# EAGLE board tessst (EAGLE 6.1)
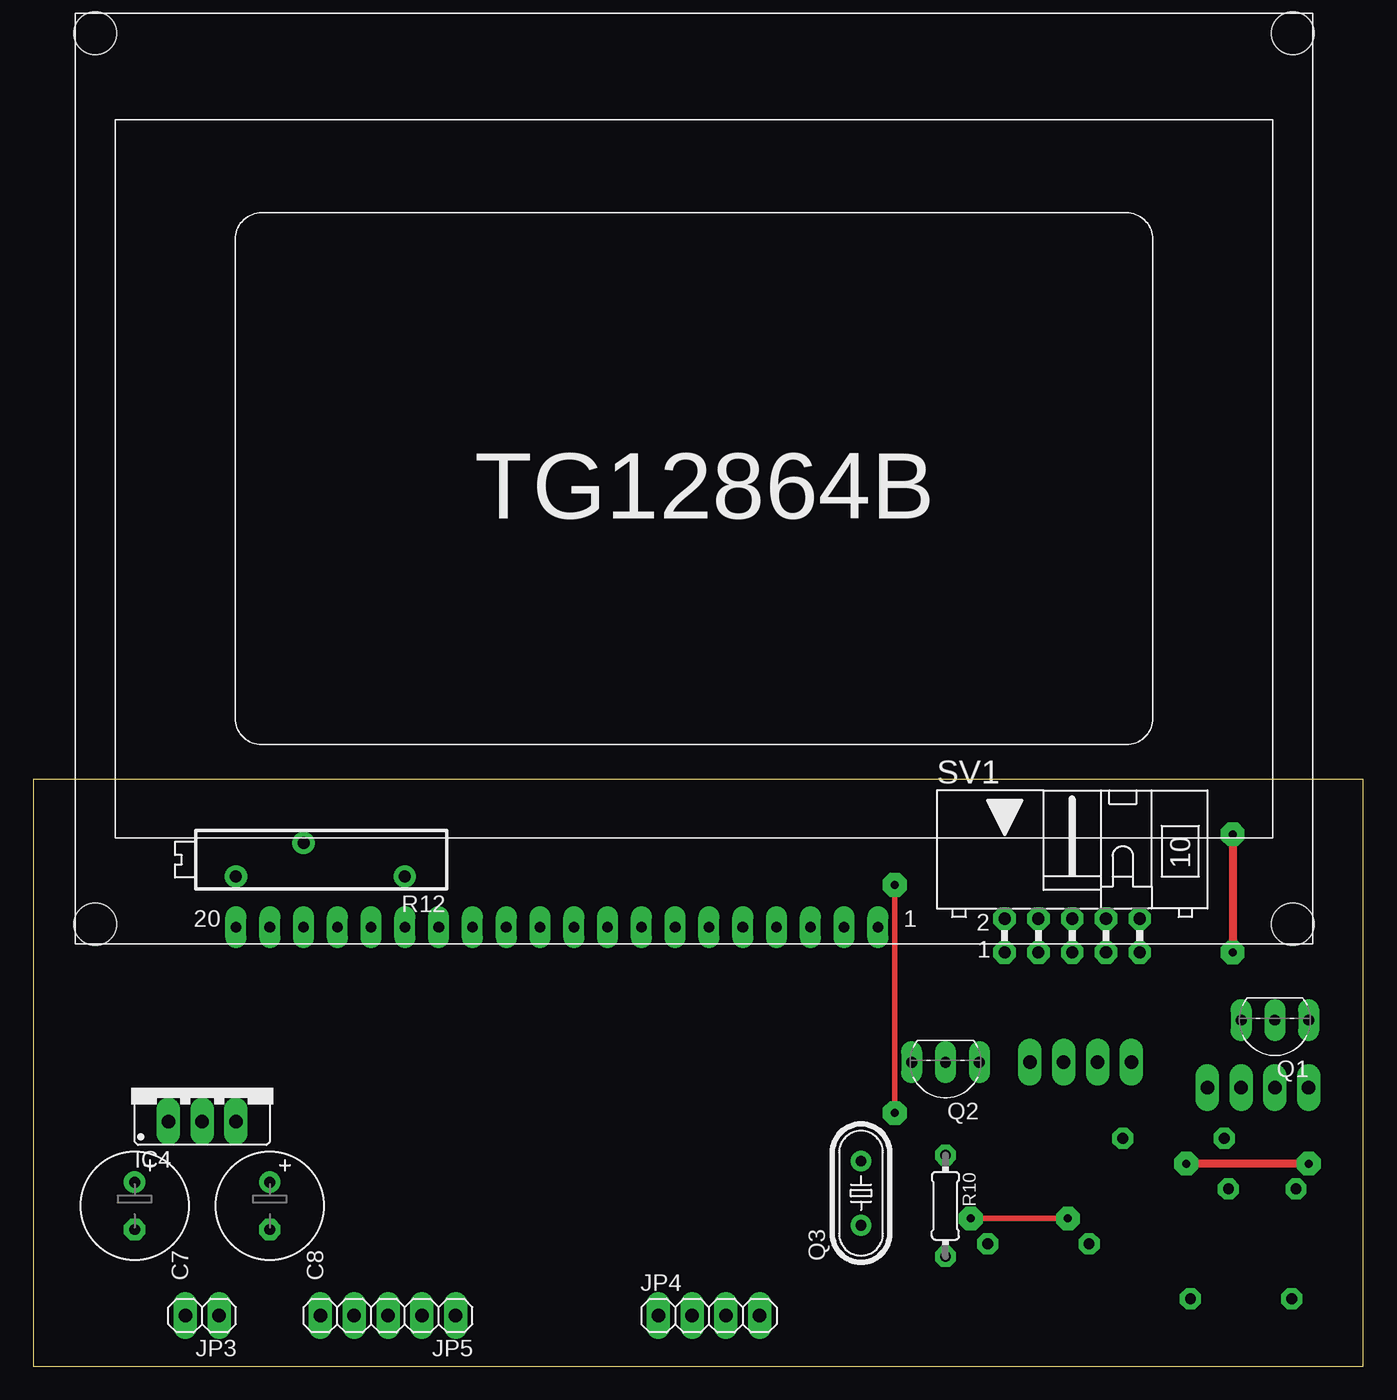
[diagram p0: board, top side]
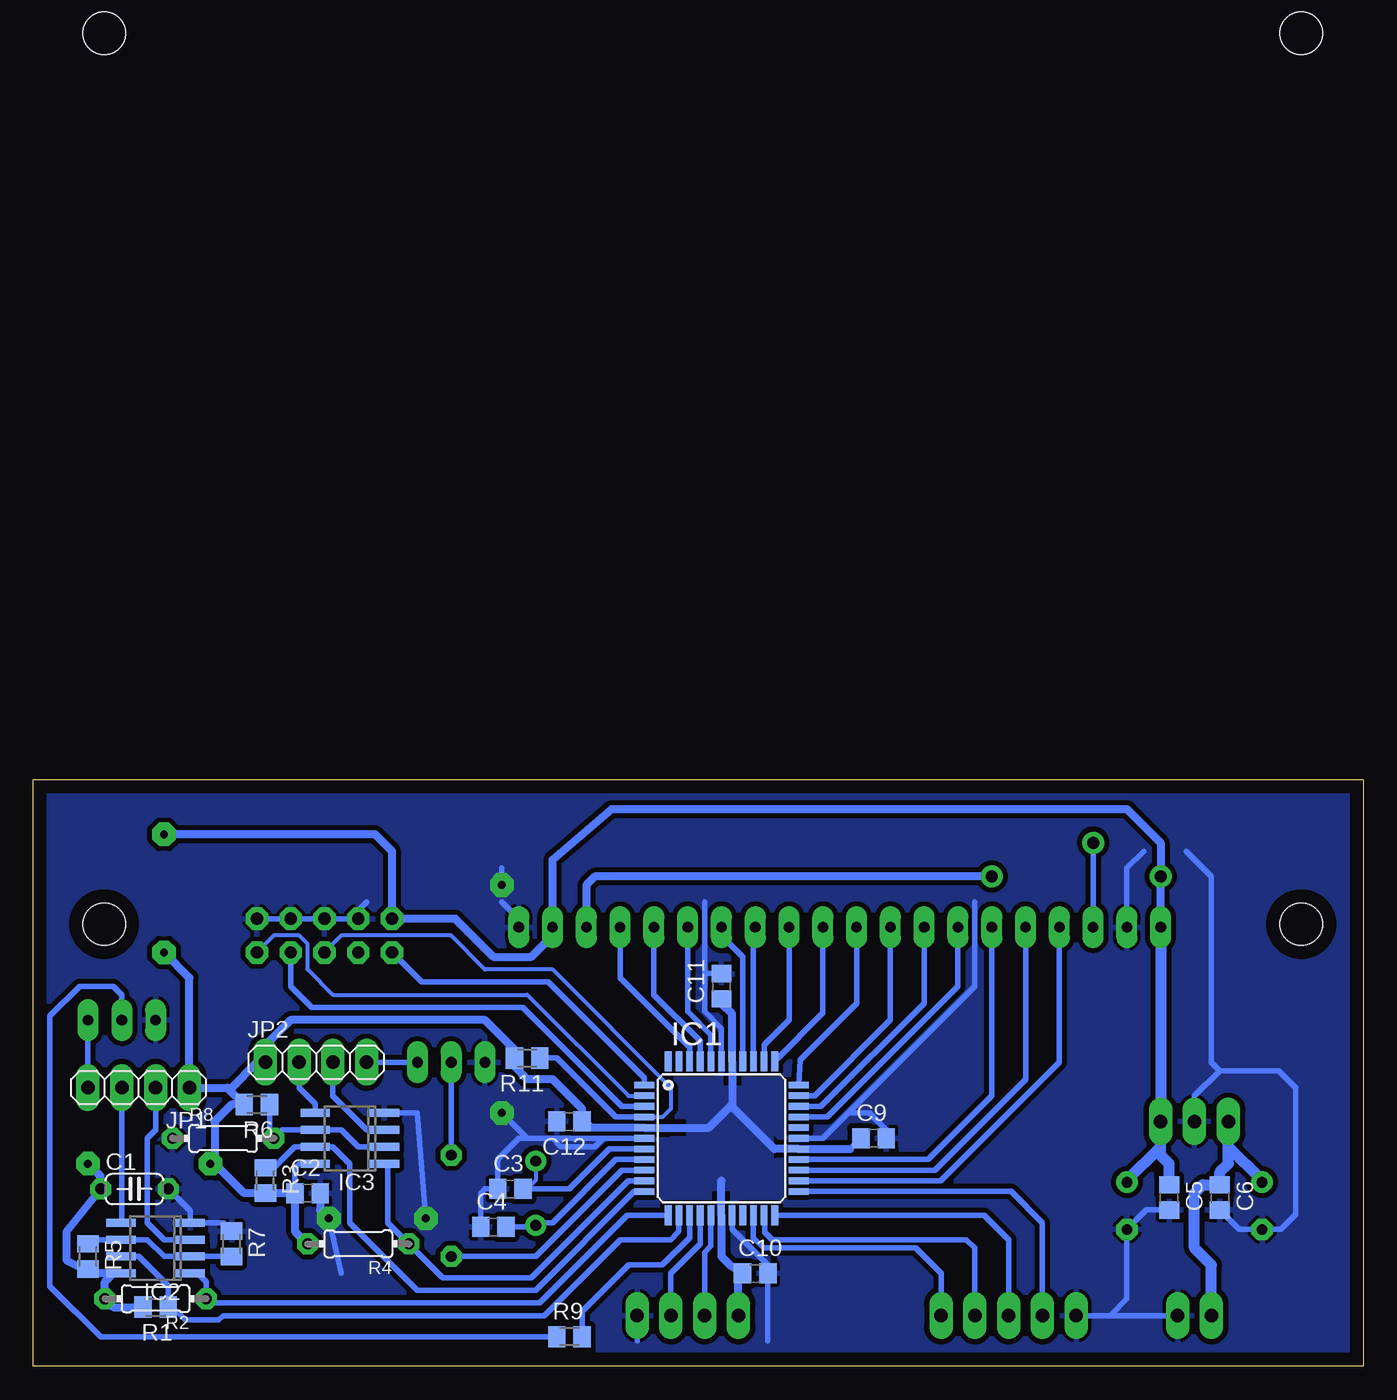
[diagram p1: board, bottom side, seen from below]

Size 100 x 44.12 mm. Coordinates in mm from the lower left corner, seen from the top.
Outline: 0,0 100,0 100,44.12 0,44.12 0,0
Copper layers (1*16): Top 0.035mm / dielectric 1.5mm / Bottom 0.035mm
Design rules: minimum track width 10mil, minimum drill 24mil, track to track 15mil, track to pad 15mil, pad to pad 8mil, via to via 8mil, smd to smd 8mil, copper to edge 40mil, drill to drill 8mil, minimum pad ring 15mil, minimum via ring 15mil, stop-mask expansion 4mil, vias tented up to drill 0mil, thermal gap 10mil

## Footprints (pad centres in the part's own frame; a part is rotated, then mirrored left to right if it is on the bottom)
C050-024X044 = drill 0.813 octagon: 1 -2.54,0; 2 2.54,0
C0805 = smd 1.3 x 1.5: 1 -0.95,0; 2 0.95,0
E3,5-8 = drill 0.813 pad 1.6: + -1.778,0 | drill 0.813 pad 1.6 octagon: - 1.778,0
TQFP44 = smd 1.5 x 0.5: 1 -5.8,4; 2 -5.8,3.2; 3 -5.8,2.4; 4 -5.8,1.6; 5 -5.8,0.8; 6 -5.8,0; 7 -5.8,-0.8; 8 -5.8,-1.6; 9 -5.8,-2.4; 10 -5.8,-3.2; 11 -5.8,-4; 23 5.8,-4; 24 5.8,-3.2; 25 5.8,-2.4; 26 5.8,-1.6; 27 5.8,-0.8; 28 5.8,0; 29 5.8,0.8; 30 5.8,1.6; 31 5.8,2.4; 32 5.8,3.2; 33 5.8,4 | smd 0.5 x 1.5: 12 -4,-5.8; 13 -3.2,-5.8; 14 -2.4,-5.8; 15 -1.6,-5.8; 16 -0.8,-5.8; 17 0,-5.8; 18 0.8,-5.8; 19 1.6,-5.8; 20 2.4,-5.8; 21 3.2,-5.8; 22 4,-5.8; 34 4,5.8; 35 3.2,5.8; 36 2.4,5.8; 37 1.6,5.8; 38 0.8,5.8; 39 0,5.8; 40 -0.8,5.8; 41 -1.6,5.8; 42 -2.4,5.8; 43 -3.2,5.8; 44 -4,5.8
SO08 = smd 0.6 x 2.2: 1 -1.905,-2.6; 2 -0.635,-2.6; 3 0.635,-2.6; 4 1.905,-2.6; 5 1.905,2.6; 6 0.635,2.6; 7 -0.635,2.6; 8 -1.905,2.6
78XXS = drill 1.016 long: GND 0,-2.54; IN -2.54,-2.54; OUT 2.54,-2.54
1X04 = drill 1.016 long: 1 -3.81,0; 2 -1.27,0; 3 1.27,0; 4 3.81,0
1X02 = drill 1.016 long: 1 -1.27,0; 2 1.27,0
1X05 = drill 1.016 long: 1 -5.08,0; 2 -2.54,0; 3 0,0; 4 2.54,0; 5 5.08,0
TO92-EBC = drill 0.813 long: B 0,-1.27; C -2.54,-1.27; E 2.54,-1.27
HC49/S = drill 0.813: 1 -2.413,0; 2 2.413,0
M0805 = smd 1.3 x 1.6: 1 -0.95,0; 2 0.95,0
0204/7 = drill 0.813 octagon: 1 -3.81,0; 2 3.81,0
RTRIMT18 = drill 0.9: 1 -7.62,1.27; 2 0,-1.27; 3 5.08,1.27
ML10L = drill 0.914 octagon: 1 -5.08,-1.27; 2 -5.08,1.27; 3 -2.54,-1.27; 4 -2.54,1.27; 5 0,-1.27; 6 0,1.27; 7 2.54,-1.27; 8 2.54,1.27; 9 5.08,-1.27; 10 5.08,1.27
TG12864B = drill 0.8 long: /RST 19.685,1.27; CS1 24.765,1.27; CS2 22.225,1.27; D/I 52.705,1.27; DB0 45.085,1.27; DB1 42.545,1.27; DB2 40.005,1.27; DB3 37.465,1.27; DB4 34.925,1.27; DB5 32.385,1.27; DB6 29.845,1.27; DB7 27.305,1.27; E 47.625,1.27; LED+ 12.065,1.27; LED- 14.605,1.27; R/W 50.165,1.27; V0 55.245,1.27; VDD 57.785,1.27; VEE 17.145,1.27; VSS 60.325,1.27 | hole 3.2: 1.5,68.5; 91.5,68.5; 91.5,1.5; 1.5,1.5

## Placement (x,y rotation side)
C1  100n  [C050-024X044]  92.39,13.34 0 bottom
C2  100n  [C0805]  79.38,13.02 0 bottom
C3  22p  [C0805]  64.14,13.34 0 bottom
C4  22p  [C0805]  65.41,10.48 0 bottom
C5  100n  [C0805]  14.61,12.7 270 bottom
C6  100n  [C0805]  10.79,12.7 270 bottom
C7  100u  [E3,5-8]  7.62,12.07 270 top
C8  100u  [E3,5-8]  17.78,12.07 270 top
C9  100n  [C0805]  36.83,17.14 0 bottom
C10  100n  [C0805]  45.72,6.99 0 bottom
C11  100n  [C0805]  48.26,28.57 90 bottom
C12  100n  [C0805]  59.69,18.41 180 bottom
IC1  MEGA32-A  [TQFP44]  48.26,17.14 0 bottom
IC2  LM393D  [SO08]  90.81,8.89 90 bottom
IC3  LM393D  [SO08]  76.2,17.14 90 bottom
IC4  [78XXS]  12.7,20.95 0 top
JP1  [1X04]  92.08,20.95 180 bottom
JP2  [1X04]  78.74,22.86 0 bottom
JP3  [1X02]  12.7,3.81 180 top
JP4  [1X04]  50.8,3.81 0 top
JP5  [1X05]  26.67,3.81 180 top
Q1  BC548  [TO92-EBC]  93.34,24.77 180 top
Q2  BC548  [TO92-EBC]  68.58,21.59 180 top
Q3  16M  [HC49/S]  62.23,13.02 90 top
R1  3k3  [M0805]  90.81,4.45 180 bottom
R2  3k3  [0204/7]  90.81,5.08 180 bottom
R3  3k3  [M0805]  82.55,13.97 270 bottom
R4  3k3  [0204/7]  75.56,9.21 180 bottom
R5  22k  [M0805]  95.89,8.25 270 bottom
R6  22k  [M0805]  83.19,19.68 180 bottom
R7  3k3  [M0805]  85.09,9.21 270 bottom
R8  3k3  [0204/7]  85.72,17.14 0 bottom
R9  22k  [M0805]  59.69,2.22 0 bottom
R10  22k  [0204/7]  68.58,12.07 270 top
R11  10k  [M0805]  62.87,23.18 180 bottom
R12  [RTRIMT18]  20.32,38.1 180 top
SV1  [ML10L]  78.11,32.38 0 top
U$1  TG12864B  [TG12864B]  3.17,31.75 0 top

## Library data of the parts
C1-C12 R1-R12 = rcl
IC1 = atmel; MPN: ATMEGA32-16AU; OC_FARNELL: 9171274; OC_NEWARK: 69K6677
IC2 IC3 = linear
IC4 = v-reg
JP1-JP5 = pinhead
Q1 Q2 = transistor-npn
Q3 = crystal; OC_FARNELL: 1667008; OC_NEWARK: unknown
SV1 = con-harting-ml; OC_FARNELL: unknown; OC_NEWARK: unknown
U$1 = TG12864B

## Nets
+5V: C1.1 C2.1 C5.1 C8.+ C9.1 C10.1 C11.1 C12.1 IC1.5 IC1.17 IC1.27 IC1.38 IC2.8 IC3.8 IC4.OUT JP1.1 JP2.1 JP4.1 R1.2 R2.2 R3.2 R4.2 R5.2 R6.2 R11.2 R12.3 SV1.2 U$1.LED+ U$1.VDD
GND: C1.2 C2.2 C3.1 C4.1 C5.2 C6.2 C7.- C8.- C9.2 C10.2 C11.2 C12.2 IC1.6 IC1.18 IC1.28 IC1.39 IC2.4 IC3.4 IC4.GND JP3.1 JP4.4 JP5.5 Q1.E Q2.E R7.1 R8.1 SV1.4 SV1.6 SV1.8 SV1.10 U$1.LED- U$1.VSS
N$1: IC1.30 U$1.DB7
N$2: IC1.31 U$1.DB6
N$3: IC1.32 U$1.DB5
N$4: IC1.33 U$1.DB4
N$5: IC1.34 U$1.DB3
N$6: IC1.35 U$1.DB2
N$7: IC1.36 U$1.DB1
N$8: IC1.37 U$1.DB0
N$9: IC1.12 IC2.1 R2.1
N$10: IC1.13 IC2.7 R1.1
N$11: IC1.11 IC3.7 R3.1
N$12: IC1.14 R9.2
N$13: IC1.10 IC3.1 R4.1
N$14: IC3.2 IC3.6 R6.1 R8.2
N$15: IC2.2 IC2.6 R5.1 R7.2
N$16: IC2.3 JP1.2
N$17: IC2.5 JP1.3
N$18: IC3.3 JP2.3
N$19: IC3.5 JP2.2
N$20: IC1.9 R10.2
N$21: JP1.4 Q1.C
N$22: Q1.B R9.1
N$23: IC1.3 SV1.7
N$24: IC1.2 SV1.9
N$25: IC1.1 SV1.1
N$26: JP2.4 Q2.C
N$27: Q2.B R10.1
N$28: IC1.4 R11.1 SV1.5
N$29: C3.2 IC1.7 Q3.2
N$30: C4.2 IC1.8 Q3.1
N$31: IC1.22 JP5.3
N$32: IC1.21 JP5.2
N$33: IC1.23 JP5.4
N$34: IC1.20 JP5.1
N$35: IC1.16 JP4.2
N$36: IC1.15 JP4.3
N$37: R12.2 U$1.VEE
N$38: R12.1 U$1.V0
N$40: IC1.42 U$1.D/I
N$41: IC1.41 U$1.R/W
N$42: IC1.40 U$1.E
N$43: IC1.26 U$1.CS1
N$44: IC1.25 U$1.CS2
N$45: IC1.24 U$1./RST
N$46: C6.1 C7.+ IC4.IN JP3.2

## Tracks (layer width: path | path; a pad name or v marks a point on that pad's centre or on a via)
+5V  (via drill 0.6, 0.6 pad 1.78)
  Top 0.61: v95.89,15.24 v86.68,15.24 | v90.17,40.01 v90.17,31.11
  Bottom 0.406: 38.58,16.34 C9.1 | C11.1 48.26,27.3 | 47.46,19.68 47.46,19.52 | IC3.8 80.01,15.24 80.33,14.92 C2.1 | 93.98,6.99 IC2.8 93.34,6.99 93.35,6.98 | 96.2,6.99 R5.2 96.2,7.3 | 82.23,13.02 R3.2 | 46.99,6.35 46.35,6.99 C10.1 46.99,6.99 | 57.95,17.95 58.42,18.41 | 63.81,22.54 R11.2 63.81,23.81 | U$1.VDD 60.96,32.38
  Bottom 0.61: 38.58,16.34 IC1.27 44.28,16.34 47.46,19.52 | 48.26,27.3 47.46,26.5 IC1.38 47.46,19.68 49.2,17.95 IC1.5 57.95,17.95 | 48.26,13.97 IC1.17 48.26,8.25 47.62,7.62 C10.1 | U$1.LED+ R12.3 15.24,39.37 17.78,41.91 56.52,41.91 60.96,38.1 U$1.VDD | C2.1 R3.2 | 96.2,6.99 93.98,6.99 94.61,6.35 R2.2 93.98,4.45 R1.2 | 96.2,7.3 97.47,7.94 97.47,10.16 C1.1 94.93,14.29 v95.89,15.24 | JP4.1 46.99,6.35 | 58.42,18.41 C12.1 58.74,19.37 60.96,21.59 62.87,21.59 63.81,22.54 | 63.81,23.81 66.04,26.04 80.64,26.04 82.55,24.13 JP2.1 83.19,22.86 85.09,20.95 85.41,20.95 | C2.1 80.33,10.16 R4.2 | 60.96,32.38 62.55,30.8 65.41,30.8 68.26,33.66 SV1.2 73.03,38.73 74.3,40.01 v90.17,40.01 | v90.17,31.11 88.27,29.21 JP1.1 85.41,20.95 | 85.41,20.95 R6.2 85.09,19.68 86.36,18.41 86.36,15.24 | R3.2 84.14,13.02 86.04,14.92 86.36,15.24 | v86.68,15.24 86.36,15.24
  Bottom 0.813: U$1.LED+ IC4.OUT 15.24,16.51 | C5.1 14.61,15.24 15.24,15.88 15.24,16.51 | C8.+ 17.78,13.97 15.24,16.51
  pour Bottom: 44.45,20.95 50.8,20.95 50.8,17.14 52.07,17.14 52.07,13.34 44.45,13.34
GND  (via drill 0.6, 0.6 pad 1.78)
  Top 0.406: v70.48,11.11 v77.79,11.11 | v64.77,19.05 v64.77,36.2
  Bottom 0.406: R7.1 85.72,10.8 IC2.4 88.2,11.69 C1.2 | SV1.10 SV1.8 SV1.6 SV1.4 76.2,33.66 74.93,34.92 | JP3.1 JP5.5 19.05,3.81 17.78,5.08 C8.- 16.32,11.75 C5.2 | C6.2 9.33,10.29 C7.- 6.22,10.29 5.08,11.43 5.08,20.95 6.35,22.22 10.79,22.22 | IC4.GND 12.7,20.32 10.79,22.22 | U$1.LED- 17.78,37.46 16.51,38.73 | 13.34,38.73 11.43,36.83 11.43,22.86 10.79,22.22 | IC1.18 47.46,10.31 44.77,7.62 C10.2 44.77,1.91 | JP4.4 54.61,1.91 | 49.53,29.53 49.53,26.67 48.26,25.4 IC1.39 | 49.53,29.53 C11.2 | 38.73,19.05 40.64,17.14 IC1.28 | 38.73,19.05 37.15,19.05 35.88,17.78 C9.2 | U$1.VSS 63.5,33.66 64.77,34.92 | C4.1 66.36,13.02 66.04,13.34 C3.1 65.08,15.56 63.5,17.14 60.96,17.14 60.33,16.51 57.78,16.51 57.15,17.14 IC1.6 62.87,17.14 v64.77,19.05 | IC3.4 71.12,19.05 v70.48,11.11 | v77.79,11.11 76.83,6.99 | 49.53,29.53 49.53,34.92 | 38.73,19.05 29.21,28.57 29.21,34.92 | v64.77,36.2 64.77,37.46
  Bottom 0.61: C2.2 78.42,11.75 v77.79,11.11
  pour Bottom: -0.64,45.09 100.97,45.09 100.97,-0.63 -0.64,-0.63
N$1
  Bottom 0.406: IC1.30 40.31,18.74 30.48,28.57 U$1.DB7
N$2
  Bottom 0.406: IC1.31 40.78,19.54 33.02,27.3 U$1.DB6
N$3
  Bottom 0.406: IC1.32 41.25,20.34 35.56,26.04 U$1.DB5
N$4
  Bottom 0.406: IC1.33 42.35,23.05 38.1,27.3 U$1.DB4
N$5
  Bottom 0.406: U$1.DB3 40.64,26.56 IC1.34
N$6
  Bottom 0.406: IC1.35 45.06,24.15 43.18,26.04 U$1.DB2
N$7
  Bottom 0.406: IC1.36 45.86,32.88 U$1.DB1
N$8
  Bottom 0.406: IC1.37 46.66,30.79 48.26,32.38 U$1.DB0
N$9
  Bottom 0.406: IC1.12 55.33,11.34 61.91,4.76 86.68,4.76 R2.1 87,6.35 87.63,6.99 IC2.1 88.27,6.92
N$10
  Bottom 0.406: IC2.7 92.08,8.25 89.86,6.04 | IC1.13 51.46,10.13 52.07,9.53 55.88,9.53 61.59,3.81 85.72,3.81 86.04,3.49 88.58,3.49 89.53,4.45 R1.1 89.86,6.04 | 89.85,6.03 89.86,6.04
N$11
  Bottom 0.406: IC1.11 54.8,13.14 62.23,5.71 71.12,5.71 76.2,10.8 76.2,15.24 77.47,16.51 IC3.7 80.33,16.51 81.92,14.92 R3.1
N$12
  Bottom 0.406: IC1.14 50.66,9.66 52.7,7.62 55.24,7.62 58.74,4.13 R9.2
N$13
  Bottom 0.406: IC1.10 55.27,13.95 62.55,6.67 69.22,6.67 R4.1 73.34,10.8 73.34,14.98 IC3.1
N$14
  Bottom 0.406: IC3.2 75.56,16.51 76.83,17.78 IC3.6 81.28,17.78 R8.2 82.23,17.46 R6.1
N$15
  Bottom 0.406: R5.1 96.2,9.53 IC2.6 91.44,9.53 90.17,8.25 IC2.2 R7.2
N$16
  Bottom 0.406: IC2.3 90.17,9.53 91.44,10.8 91.44,17.14 90.81,17.78 JP1.2
N$17
  Bottom 0.406: 93.98,10.8 IC2.5 93.34,10.86 JP1.3
N$18
  Bottom 0.406: IC3.3 74.93,17.78 77.47,20.32 JP2.3
N$19
  Bottom 0.406: IC3.5 78.8,19.74 80.01,20.95 JP2.2
N$20
  Bottom 0.406: IC1.9 55.74,14.75 62.23,8.25 R10.2
N$21
  Bottom 0.406: JP1.4 Q1.C
N$22
  Bottom 0.406: 93.67,26.36 Q1.B 93.34,27.94 93.98,28.57 96.52,28.57 98.74,26.35 98.74,6.03 94.93,2.22 R9.1
N$23
  Bottom 0.406: IC1.3 55.74,19.54 63.18,26.99 79.06,26.99 80.64,28.57 SV1.7
N$24
  Bottom 0.305: 54.03,20.32 55.24,20.32 62.87,27.94 77.47,27.94 79.38,29.84 79.38,31.75 80.01,32.38 81.92,32.38 SV1.9
  Bottom 0.406: 53.98,20.32 54.03,20.32 IC1.2
N$25
  Bottom 0.406: IC1.1 54.06,21.68 61.28,28.89 70.8,28.89 SV1.1
N$26
  Bottom 0.406: JP2.4 Q2.C
N$27
  Bottom 0.406: R10.1 Q2.B
N$28
  Bottom 0.305: 54.05,18.73 52.7,18.73 52.07,19.37 52.07,20.95 60.96,29.84 66.04,29.84 68.58,32.38 76.83,32.38 SV1.5
  Bottom 0.406: 54.05,18.73 IC1.4 56.21,18.74 60.64,23.18 R11.1
N$29
  Bottom 0.305: 62.23,15.24 62.23,13.97 62.87,13.34
  Bottom 0.406: IC1.7 56.68,16.34 59.69,13.34 62.87,13.34 C3.2 | 62.23,15.24 Q3.2
N$30
  Bottom 0.406: C4.2 62.55,10.48 62.42,10.61 | 62.42,10.61 62.23,10.8 | 62.42,10.61 Q3.1 62.04,10.8 60.96,10.8 56.21,15.55 IC1.8
N$31
  Bottom 0.406: IC1.22 28.49,11.34 26.67,9.53 JP5.3
N$32
  Bottom 0.406: IC1.21 45,11.34 45,10.07 44.45,9.53 29.84,9.53 29.21,8.89 JP5.2
N$33
  Bottom 0.406: IC1.23 26.48,13.14 24.13,10.8 JP5.4
N$34
  Bottom 0.406: JP5.1 31.75,6.99 33.66,8.89 45.09,8.89 45.86,9.66 IC1.20
N$35
  Bottom 0.406: IC1.16 49.06,9.04 49.53,8.57 JP4.2
N$36
  Bottom 0.406: IC1.15 49.86,9.2 52.07,6.99 JP4.3
N$37
  Bottom 0.406: U$1.VEE R12.2
N$38
  Bottom 0.61: R12.1 57.78,36.83 58.42,36.2 U$1.V0
N$40
  Bottom 0.406: IC1.42 50.66,23.99 55.88,29.21 U$1.D/I
N$41
  Bottom 0.406: IC1.41 49.86,24.46 53.34,27.94 U$1.R/W
N$42
  Bottom 0.406: IC1.40 49.06,24.93 50.8,26.67 U$1.E
N$43
  Bottom 0.406: IC1.26 32.72,15.55 27.94,20.32 U$1.CS1
N$44
  Bottom 0.406: IC1.25 32.24,14.75 25.4,21.59 U$1.CS2
N$45
  Bottom 0.406: IC1.24 31.77,13.95 22.86,22.86 U$1./RST
N$46
  Bottom 0.813: 10.16,16.51 10.16,15.24 10.79,14.61 C6.1 12.06,13.65 12.7,13.02 12.7,8.89 11.43,7.62 JP3.2 | 10.16,16.51 IC4.IN | C7.+ 7.62,13.97 10.16,16.51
